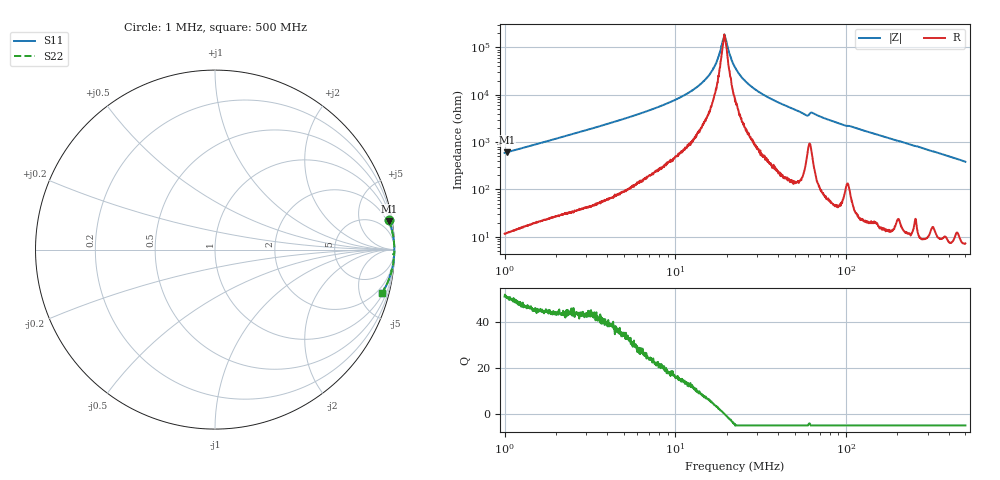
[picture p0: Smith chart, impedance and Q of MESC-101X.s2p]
!s-Parameter Generated by FASTRON Sdn. Bhd.
!FASTRON P/N : MESC-101X
!Keysight Technologies,E4991B,MY54100416,A.01.15
!Date: Fri Mar 27 09:57:55 2026
!Version  : Rev00 Fri Mar 27 09:57:55 2026
!Data & Calibration Information:
!PortZ  Port1:50+j0  Port2:50+j0
!When reading, reference impedance value at option line is always used.
!Remarks : This data is being provided solely for informational purposes.
!Freq	S11	S21	S12	S22
# Hz S dB R 50
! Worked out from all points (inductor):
!   1601 points, 1 MHz to 500 MHz, reference 50 ohm
!   read as one part in series: L = 93.5 uH near 1.032 MHz
!   highest Q = 50.8 at 1.032 MHz (marker M1), where L = 94.1 uH
!   self-resonance near 19.37 MHz
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1000000  -0.15 9.6  -15.59 -79.3  -15.59 -79.3  -0.15 9.6
1031561  -0.14 9.3  -15.85 -79.6  -15.85 -79.6  -0.14 9.3
2820919  -0.03 3.4  -24.51 -85.3  -24.51 -85.3  -0.03 3.4
7957584  -0.01 1.0  -34.84 -86.2  -34.84 -86.2  -0.01 1.0
1.168907e7  -0.01 0.5  -40.46 -85.1  -40.46 -85.1  -0.01 0.5
1.469957e7  -0.01 0.3  -45.81 -81.8  -45.81 -81.8  -0.01 0.3
1.588699e7  -0.01 0.2  -48.60 -80.4  -48.60 -80.4  -0.01 0.2
1.703747e7  -0.01 0.1  -52.31 -75.2  -52.31 -75.2  -0.01 0.1
1.791984e7  -0.01 0.1  -56.23 -68.0  -56.23 -68.0  -0.01 0.1
1.892127e7  -0.00 0.0  -62.72 -40.2  -62.72 -40.2  -0.00 0.0
1.93674e7  -0.00 0.0  -65.50 -4.3  -65.50 -4.3  -0.00 0.0
1.982405e7  -0.00 -0.0  -63.16 35.9  -63.16 35.9  -0.00 -0.0
2.117722e7  -0.01 -0.1  -55.58 68.3  -55.58 68.3  -0.01 -0.1
2.236068e7  -0.00 -0.1  -51.62 78.9  -51.62 78.9  -0.00 -0.1
2.397996e7  -0.00 -0.2  -48.21 81.6  -48.21 81.6  -0.00 -0.2
2.55175e7  -0.00 -0.3  -45.99 83.9  -45.99 83.9  -0.00 -0.3
3.246558e7  -0.00 -0.6  -40.22 86.7  -40.22 86.7  -0.00 -0.6
5.79115e7  -0.02 -1.5  -31.54 83.5  -31.54 83.5  -0.02 -1.5
6.307767e7  -0.03 -1.3  -32.48 80.9  -32.48 80.9  -0.03 -1.3
9.632587e7  -0.02 -2.5  -27.30 86.0  -27.30 86.0  -0.02 -2.5
1.77937e8  -0.04 -4.7  -21.73 84.7  -21.73 84.7  -0.04 -4.7
5e8  -0.32 -14.5  -12.02 74.4  -12.02 74.4  -0.32 -14.5
